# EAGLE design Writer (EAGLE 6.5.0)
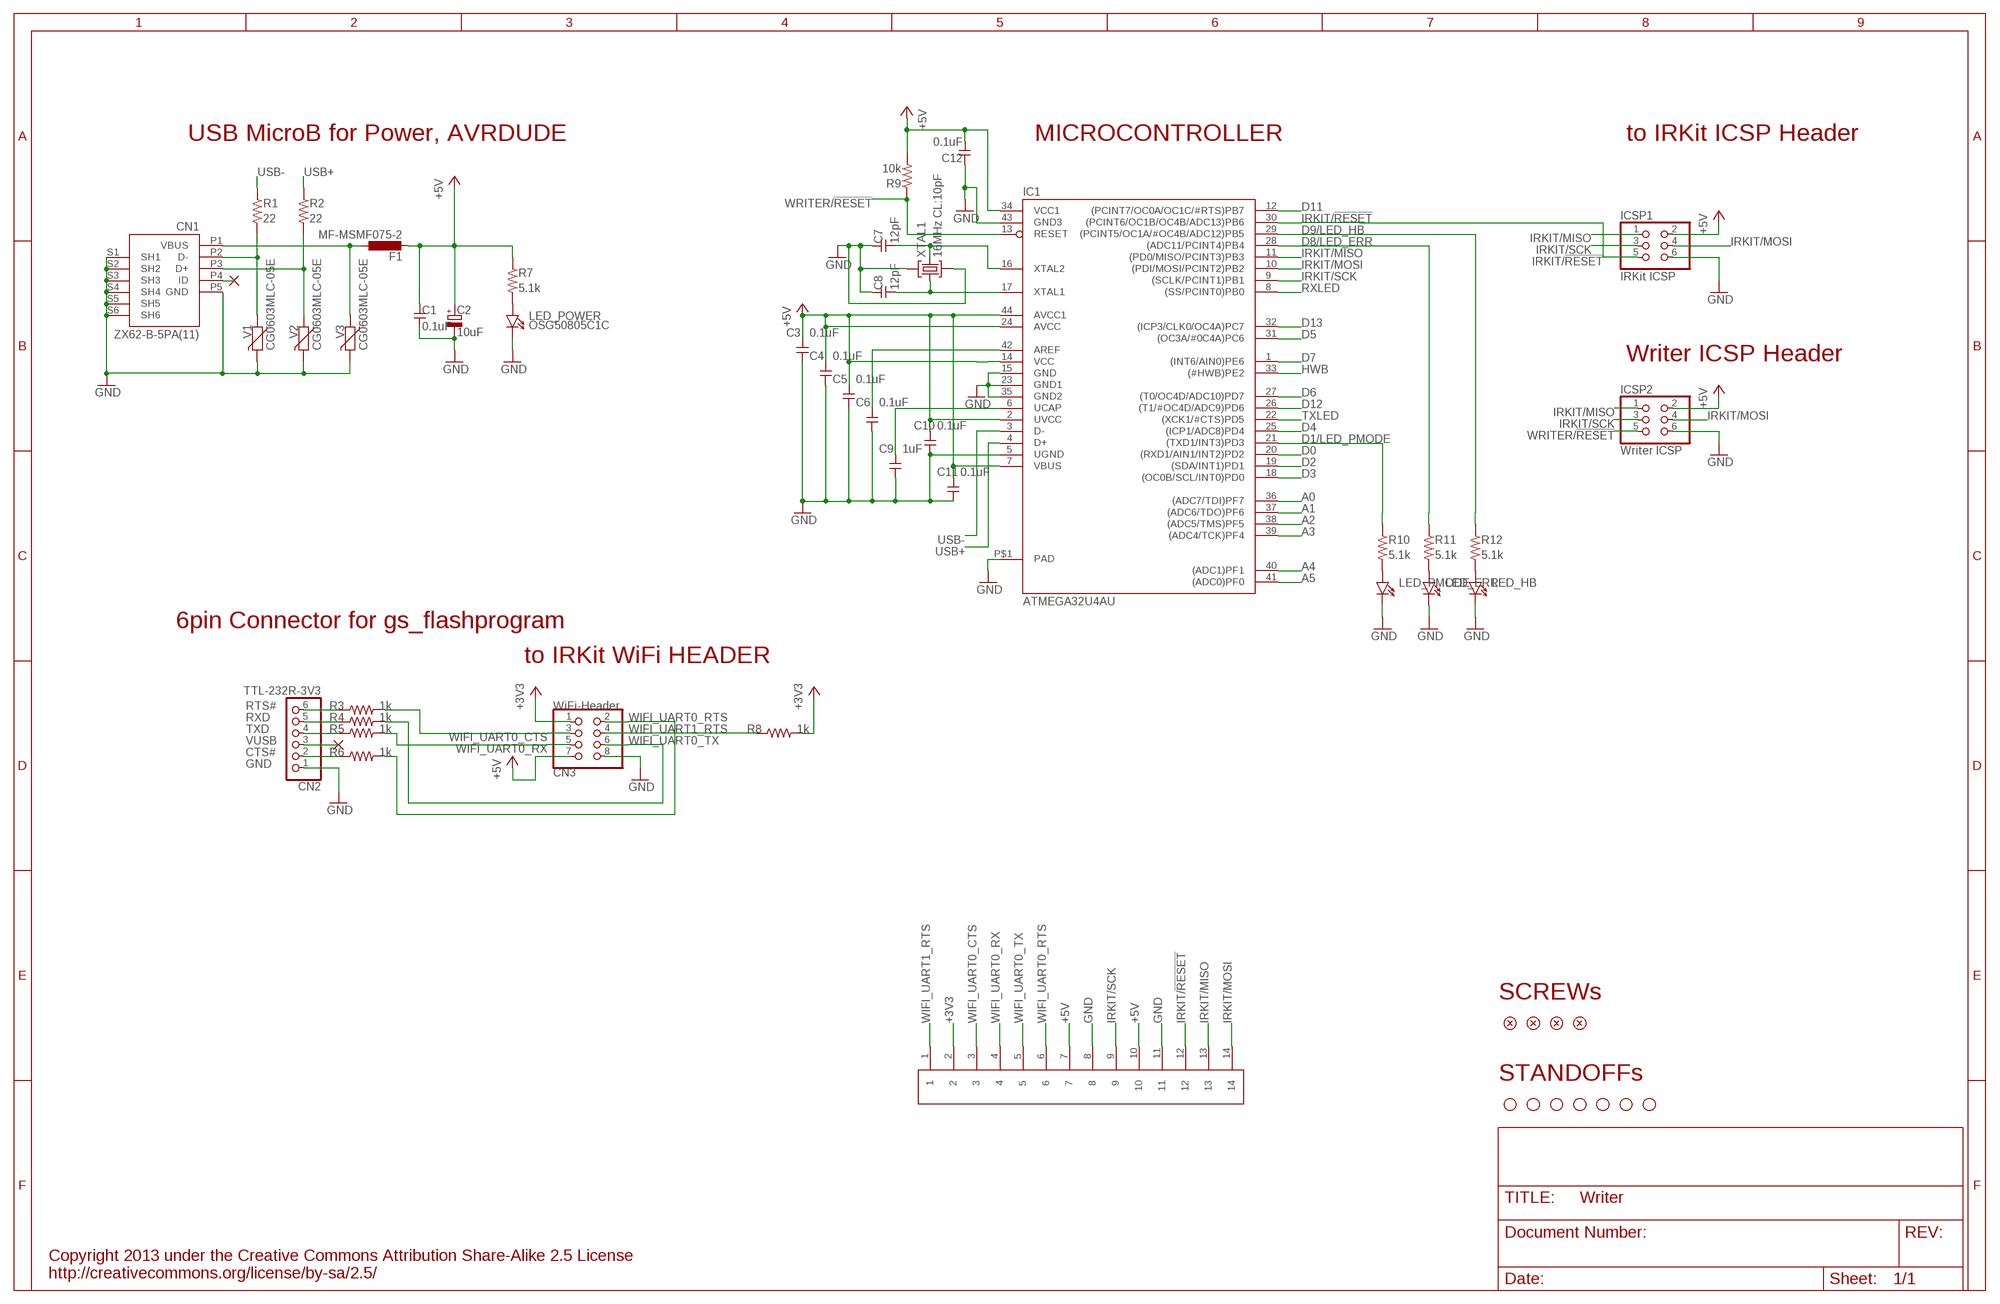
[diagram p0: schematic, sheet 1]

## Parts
C1  0.1uF  CAPACITOR2012  [SMD2012]
C2  10uF  CAPACITOR-POLPANASONIC_B  [PANASONIC_B]
C3  0.1uF  CAPACITOR2012  [SMD2012]
C4  0.1uF  CAPACITOR2012  [SMD2012]
C5  0.1uF  CAPACITOR2012  [SMD2012]
C6  0.1uF  CAPACITOR2012  [SMD2012]
C7  12pF  CAPACITOR2012  [SMD2012]
C8  12pF  CAPACITOR2012  [SMD2012]
C9  1uF  CAPACITOR2012  [SMD2012]
C10  0.1uF  CAPACITOR2012  [SMD2012]
C11  0.1uF  CAPACITOR2012  [SMD2012]
C12  0.1uF  CAPACITOR2012  [SMD2012]
CN1  ZX62-B-5PA(11)  USB-CONNECTORMICROB  [USB-MICROB]
CN2  TTL-232R-3V3  PINHD-1X6/90  [1X06/90]
CN3  WiFi-Header  PINHD-2X4/D1.1  [2X04/D1.1]
CN4  SOCKET-HEADER-7614-5002  [SOCKET-HEADER-7614-5002]
F1  MF-MSMF075-2  L-EUL1812  [L1812]
IC1  ATMEGA32U4AU  [TQFP44-PAD]
ICSP1  IRKit ICSP  PINHD-2X3/D1.1  [2X03/D1.1]
ICSP2  Writer ICSP  PINHD-2X3  [2X03]
LED_ERR  LED-2012  [LED2012]
LED_HB  LED-2012  [LED2012]
LED_PMODE  LED-2012  [LED2012]
LED_POWER  OSG50805C1C  LED-2012  [LED2012]
R1  22  RESISTOR-US2012  [SMD2012]
R2  22  RESISTOR-US2012  [SMD2012]
R3  1k  RESISTOR-US2012  [SMD2012]
R4  1k  RESISTOR-US2012  [SMD2012]
R5  1k  RESISTOR-US2012  [SMD2012]
R6  1k  RESISTOR-US2012  [SMD2012]
R7  5.1k  RESISTOR-US2012  [SMD2012]
R8  1k  RESISTOR-US2012  [SMD2012]
R9  10k  RESISTOR-US2012  [SMD2012]
R10  5.1k  RESISTOR-US2012  [SMD2012]
R11  5.1k  RESISTOR-US2012  [SMD2012]
R12  5.1k  RESISTOR-US2012  [SMD2012]
SCREW1  flat-head M3 self-tapping  SCREW  [SCREW-M3]
SCREW2  flat-head M3 self-tapping  SCREW  [SCREW-M3]
SCREW3  flat-head M3 self-tapping  SCREW  [SCREW-M3]
SCREW4  flat-head M3 self-tapping  SCREW  [SCREW-M3]
STANDOFF1  STAND-OFF  [STAND-OFF]
STANDOFF2  STAND-OFF  [STAND-OFF]
STANDOFF3  STAND-OFF  [STAND-OFF]
STANDOFF4  STAND-OFF  [STAND-OFF]
STANDOFF5  STAND-OFF  [STAND-OFF]
STANDOFF6  STAND-OFF  [STAND-OFF]
STANDOFF7  STAND-OFF  [STAND-OFF]
V1  CG0603MLC-05E  VARISTORCN0603  [CT/CN0603]
V2  CG0603MLC-05E  VARISTORCN0603  [CT/CN0603]
V3  CG0603MLC-05E  VARISTORCN0603  [CT/CN0603]
XTAL1  16MHz CL:10pF  CRYSTAL-3.2-2.5  [CRYSTAL-3.2-2.5]

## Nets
+3V3 [3.3v]: CN3.1 CN4.2 R8.2
+5V [power]: C1.1 C2.+ C3.2 C4.2 C5.2 C10.2 C11.2 C12.2 CN3.7 CN4.7 CN4.10 F1.2 IC1.2(UVCC) IC1.7(VBUS) IC1.14(VCC) IC1.24(AVCC) IC1.34(VCC1) IC1.44(AVCC1) ICSP1.2 ICSP2.2 R7.1 R9.2
A0: IC1.36((ADC7/TDI)PF7)
A1: IC1.37((ADC6/TDO)PF6)
A2: IC1.38((ADC5/TMS)PF5)
A3: IC1.39((ADC4/TCK)PF4)
A4: IC1.40((ADC1)PF1)
A5: IC1.41((ADC0)PF0)
AREF [power]: C6.2 IC1.42(AREF)
CTS#: CN2.2 R6.1
D0: IC1.20((RXD1/AIN1/INT2)PD2)
D1/LED_PMODE: IC1.21((TXD1/INT3)PD3) R10.1
D2: IC1.19((SDA/INT1)PD1)
D3: IC1.18((OC0B/SCL/INT0)PD0)
D4: IC1.25((ICP1/ADC8)PD4)
D5: IC1.31((OC3A/#0C4A)PC6)
D6: IC1.27((T0/OC4D/ADC10)PD7)
D7: IC1.1((INT6/AIN0)PE6)
D8/LED_ERR: IC1.28((ADC11/PCINT4)PB4) R11.1
D9/LED_HB: IC1.29((PCINT5/OC1A/#OC4B/ADC12)PB5) R12.1
D11: IC1.12((PCINT7/OC0A/OC1C/#RTS)PB7)
D12: IC1.26((T1/#OC4D/ADC9)PD6)
D13: IC1.32((ICP3/CLK0/OC4A)PC7)
GND [gnd]: C1.2 C2.- C3.1 C4.1 C5.1 C6.1 C7.1 C8.1 C9.1 C10.1 C11.1 C12.1 CN1.P5(GND) CN1.S1(SH1) CN1.S2(SH2) CN1.S3(SH3) CN1.S4(SH4) CN1.S5(SH5) CN1.S6(SH6) CN2.1 CN3.8 CN4.8 CN4.11 IC1.5(UGND) IC1.15(GND) IC1.23(GND1) IC1.35(GND2) IC1.43(GND3) IC1.P$1(PAD) ICSP1.6 ICSP2.6 LED_ERR.K LED_HB.K LED_PMODE.K LED_POWER.K V1.2 V2.2 V3.2 XTAL1.2(GND) XTAL1.4(GND)
HWB: IC1.33((#HWB)PE2)
IRKIT/!RESET: CN4.12 IC1.30((PCINT6/OC1B/OC4B/ADC13)PB6) ICSP1.5
IRKIT/MISO: CN4.13 IC1.11((PD0/MISO/PCINT3)PB3) ICSP1.1 ICSP2.1
IRKIT/MOSI: CN4.14 IC1.10((PDI/MOSI/PCINT2)PB2) ICSP1.4 ICSP2.4
IRKIT/SCK: CN4.9 IC1.9((SCLK/PCINT1)PB1) ICSP1.3 ICSP2.3
N$1: LED_PMODE.A R10.2
N$2: LED_ERR.A R11.2
N$3: LED_POWER.A R7.2
N$4: LED_HB.A R12.2
N$48: CN1.P2(D-) R1.2 V1.1
N$51: CN1.P3(D+) R2.2 V2.1
N$52: CN1.P1(VBUS) F1.1 V3.1
RTS#: CN2.6 R3.1
RXD: CN2.5 R4.1
RXLED: IC1.8((SS/PCINT0)PB0)
TXD: CN2.4 R5.1
TXLED: IC1.22((XCK1/#CTS)PD5)
UCAP: C9.2 IC1.6(UCAP)
USB+: IC1.4(D+) R2.1
USB-: IC1.3(D-) R1.1
USB-ID: CN1.P4(ID)
VUSB: CN2.3
WIFI_UART0_CTS: CN3.3 CN4.3 R3.2
WIFI_UART0_RTS: CN3.2 CN4.6 R6.2
WIFI_UART0_RX: CN3.5 CN4.4 R5.2
WIFI_UART0_TX: CN3.6 CN4.5 R4.2
WIFI_UART1_RTS: CN3.4 CN4.1 R8.1
WRITER/!RESET: IC1.13(RESET) ICSP2.5 R9.1
XTAL1: C8.2 IC1.17(XTAL1) XTAL1.1(C1)
XTAL2: C7.2 IC1.16(XTAL2) XTAL1.3(C2)

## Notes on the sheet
- USB MicroB for Power, AVRDUDE | MICROCONTROLLER | to IRKit ICSP Header
- Writer ICSP Header
- 6pin Connector for gs_flashprogram
- to IRKit WiFi HEADER
- SCREWs
- STANDOFFs
- Copyright 2013 under the Creative Commons Attribution Share-Alike 2.5 License
  http://creativecommons.org/license/by-sa/2.5/

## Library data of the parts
C1 C3-C12 = my:CAPACITOR: Generic Capacitor
C2 = my:CAPACITOR-POL: Generic Capacitor with Polarity
CN1 = my:USB-CONNECTOR
CN2 = my:PINHD-1X6: PIN HEADER
CN3 = my:PINHD-2X4: PIN HEADER
CN4 = my:SOCKET-HEADER: Sumitomo Standard Socket
F1 = my:L-EU: INDUCTOR, European symbol
IC1 = my:ATMEGA32U4
ICSP1 ICSP2 = my:PINHD-2X3: PIN HEADER
LED_ERR LED_HB LED_PMODE LED_POWER = my:LED: Through-hole LED
R1-R12 = my:RESISTOR-US: Generic Registor
SCREW1-SCREW4 = my:SCREW
STANDOFF1-STANDOFF7 = my:STAND-OFF: #4 Stand Off
V1-V3 = my:VARISTOR: VARISTOR
XTAL1 = my:CRYSTAL-3.2-2.5

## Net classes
0 default: width 0.254 mm
1 power: width 0.406 mm
2 ir-power: width 0.813 mm
3 gnd: width 0.406 mm
4 3.3v: width 0.406 mm

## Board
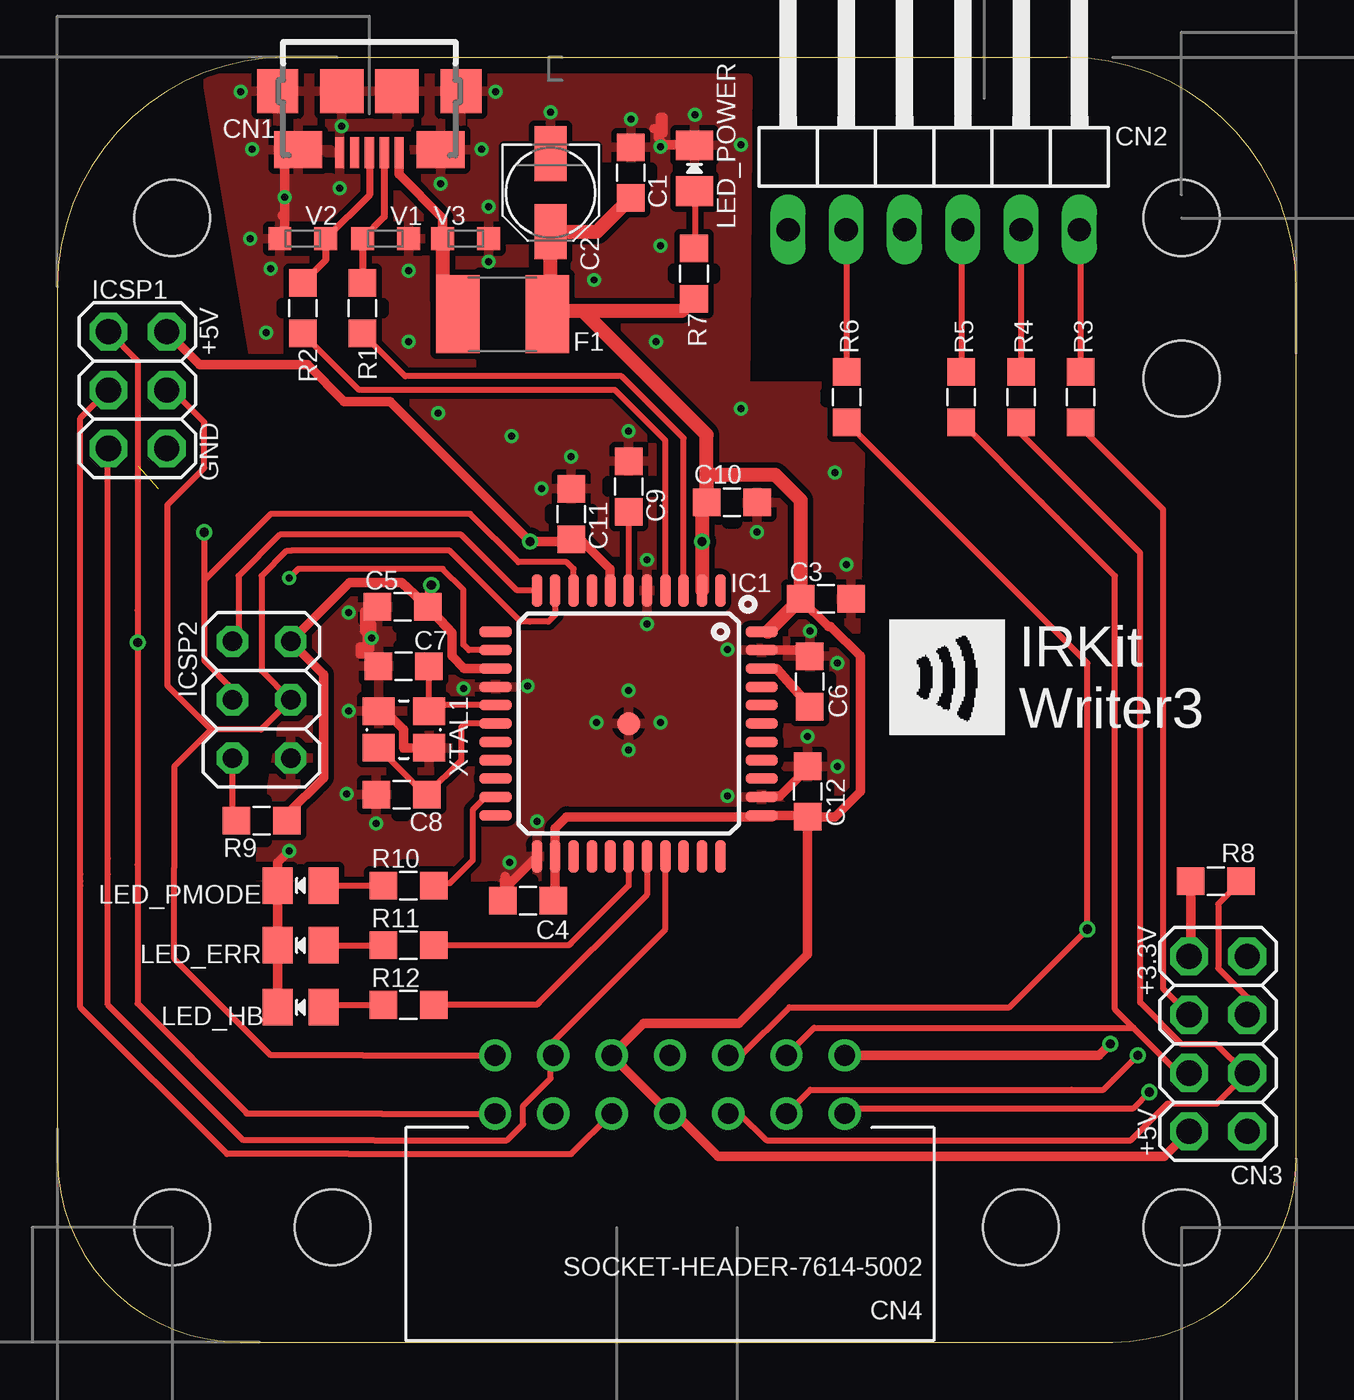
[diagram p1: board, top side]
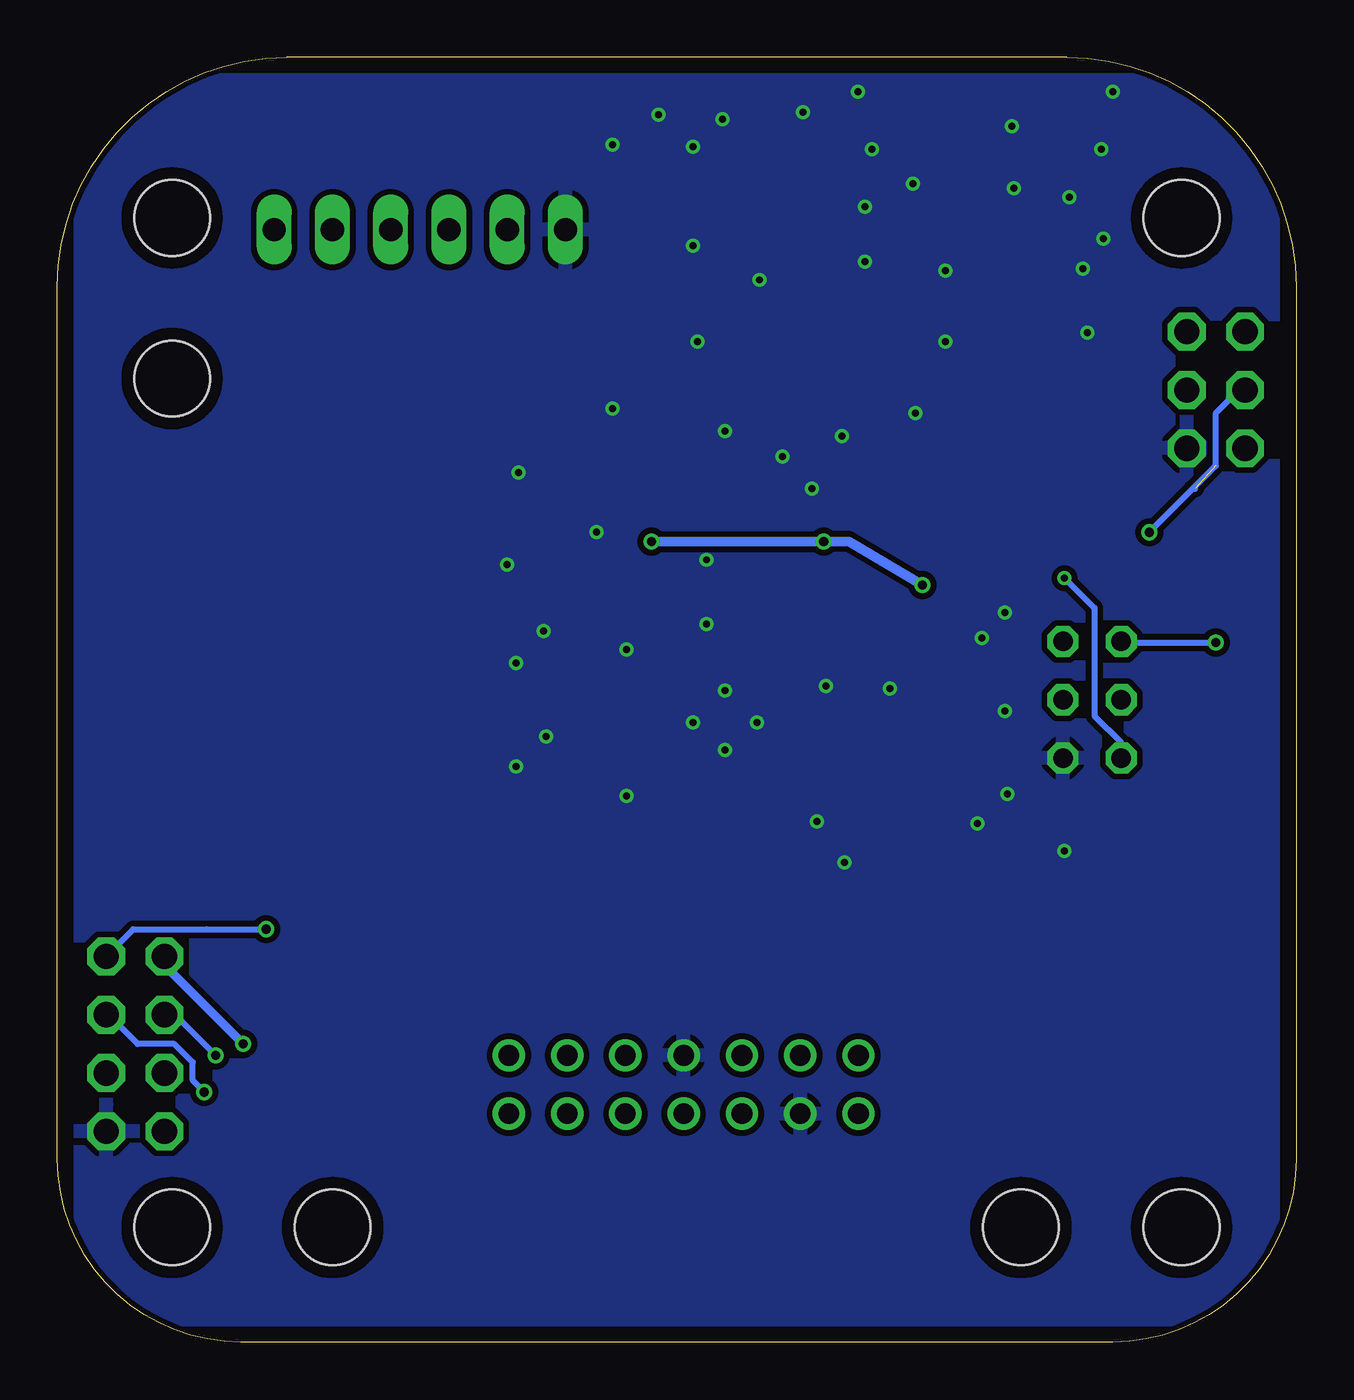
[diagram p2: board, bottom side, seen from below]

Size 54 x 56 mm. Coordinates in mm from the lower left corner, seen from the top.
Outline: 8,0 46,0 arc90 54,8 54,17.5 54,34.8 54,46 arc90 44,56 34.1,56 34,56 20,56 10,56 arc90 0,46 0,8 arc90 8,0
Copper layers (1*16): Top 0.035mm / dielectric 1.5mm / Bottom 0.035mm
Design rules "Fusion_eagle_rule_v1.1": minimum track width 6mil, minimum drill 12mil, track to track 6mil, track to pad 6mil, pad to pad 6mil, via to via 6mil, smd to smd 0mil, copper to edge 10mil, drill to drill 10mil, minimum pad ring 10mil, minimum via ring 6mil, stop-mask expansion 2mil, vias tented up to drill 100mil, thermal gap 10mil

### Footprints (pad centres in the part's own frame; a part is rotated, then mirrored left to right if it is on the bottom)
SMD2012 = smd 1.2 x 1.2: 1 -1.1,0; 2 1.1,0
PANASONIC_B = smd 2.4 x 1.4: + 1.7,0; - -1.7,0
USB-MICROB = smd 0.4 x 1.35: P1 -1.3,2.675; P2 -0.65,2.675; P3 0,2.675; P4 0.65,2.675; P5 1.3,2.675 | smd 1.8 x 1.9: S1 -4,0; S2 4,0 | smd 2.1 x 1.6: S3 -3.1,2.55; S4 3.1,2.55 | smd 1.9 x 1.9: S5 -1.2,0; S6 1.2,0
1X06/90 = drill 1.016 long: 1 -6.35,-3.81; 2 -3.81,-3.81; 3 -1.27,-3.81; 4 1.27,-3.81; 5 3.81,-3.81; 6 6.35,-3.81
2X04/D1.1 = drill 1.1 octagon: 1 -3.81,-1.27; 2 -3.81,1.27; 3 -1.27,-1.27; 4 -1.27,1.27; 5 1.27,-1.27; 6 1.27,1.27; 7 3.81,-1.27; 8 3.81,1.27
SOCKET-HEADER-7614-5002 = drill 0.9: 1 -7.62,2.54; 2 -7.62,0; 3 -5.08,2.54; 4 -5.08,0; 5 -2.54,2.54; 6 -2.54,0; 7 0,2.54; 8 0,0; 9 2.54,2.54; 10 2.54,0; 11 5.08,2.54; 12 5.08,0; 13 7.62,2.54; 14 7.62,0
L1812 = smd 1.9 x 3.4: 1 -1.95,0; 2 1.95,0
TQFP44-PAD = smd 1.4 x 0.45: 1 -5.8,4; 2 -5.8,3.2; 3 -5.8,2.4; 4 -5.8,1.6; 5 -5.8,0.8; 6 -5.8,0; 7 -5.8,-0.8; 8 -5.8,-1.6; 9 -5.8,-2.4; 10 -5.8,-3.2; 11 -5.8,-4; 23 5.8,-4; 24 5.8,-3.2; 25 5.8,-2.4; 26 5.8,-1.6; 27 5.8,-0.8; 28 5.8,0; 29 5.8,0.8; 30 5.8,1.6; 31 5.8,2.4; 32 5.8,3.2; 33 5.8,4 | smd 0.45 x 1.4: 12 -4,-5.8; 13 -3.2,-5.8; 14 -2.4,-5.8; 15 -1.6,-5.8; 16 -0.8,-5.8; 17 0,-5.8; 18 0.8,-5.8; 19 1.6,-5.8; 20 2.4,-5.8; 21 3.2,-5.8; 22 4,-5.8; 34 4,5.8; 35 3.2,5.8; 36 2.4,5.8; 37 1.6,5.8; 38 0.8,5.8; 39 0,5.8; 40 -0.8,5.8; 41 -1.6,5.8; 42 -2.4,5.8; 43 -3.2,5.8; 44 -4,5.8 | smd 1 x 1: P$1 0,0
2X03/D1.1 = drill 1.1 octagon: 1 -2.54,-1.27; 2 -2.54,1.27; 3 0,-1.27; 4 0,1.27; 5 2.54,-1.27; 6 2.54,1.27
2X03 = drill 0.85 octagon: 1 -2.54,-1.27; 2 -2.54,1.27; 3 0,-1.27; 4 0,1.27; 5 2.54,-1.27; 6 2.54,1.27
LED2012 = smd 1.3 x 1.6: A -1,0; K 1,0
STAND-OFF = hole 3.302: 0,0
CT/CN0603 = smd 1 x 1: 1 -1,0; 2 1,0
CRYSTAL-3.2-2.5 = smd 1.4 x 1.2: 1 -1.1,-0.8; 2 1.1,-0.8; 3 1.1,0.8; 4 -1.1,0.8

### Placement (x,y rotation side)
C1  25,50.97 90 top
C2  21.5,50.1 270 top
C3  33.5,32.4 180 top
C4  20.51,19.25 0 top
C5  15.05,32.05 0 top
C6  32.8,28.8 270 top
C7  15.1,29.46 0 top
C8  15,23.86 0 top
C9  24.9,37.3 270 top
C10  29.4,36.6 180 top
C11  22.4,36.1 270 top
C12  32.7,24 270 top
CN1  13.6,54.52 180 top
CN2  38.2,52.3 0 top
CN3  50.6,13 270 top
CN4  26.7,12.5 180 top
F1  19.4,44.8 0 top
IC1  24.9,26.96 270 top
ICSP1  3.5,41.5 270 top
ICSP2  8.9,28 270 top
LED_ERR  10.6,17.3 180 top
LED_HB  10.6,14.6 180 top
LED_PMODE  10.6,19.9 180 top
LED_POWER  27.77,51.16 90 top
R1  13.3,45.06 90 top
R2  10.7,45.06 90 top
R3  44.6,41.2 270 top
R4  42,41.2 270 top
R5  39.4,41.2 270 top
R6  34.4,41.2 270 top
R7  27.75,46.58 90 top
R8  50.5,20.1 180 top
R9  8.9,22.73 0 top
R10  15.3,19.9 180 top
R11  15.3,17.3 180 top
R12  15.3,14.7 180 top
SCREW1  not placed on the board
SCREW2  not placed on the board
SCREW3  not placed on the board
SCREW4  not placed on the board
STANDOFF1  49,5 0 top
STANDOFF2  5,5 0 top
STANDOFF3  49,49 0 top
STANDOFF4  5,49 0 top
STANDOFF5  12,5 0 top
STANDOFF6  42,5 0 top
STANDOFF7  49,42 0 top
U$1  [IRKIT-LOGO]  36.3,26.5 0 top
V1  14.3,48.1 0 top
V2  10.7,48.1 180 top
V3  17.8,48.1 0 top
XTAL1  15.1,26.7 0 top

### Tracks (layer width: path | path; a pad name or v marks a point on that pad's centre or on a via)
+3V3  (via drill 0.4)
  Top 0.406: R8.2 49.4,16.9 CN3.1 | CN4.2 45.4,12.5 v45.9,13
  Bottom 0.406: v45.9,13 49.33,16.43 CN3.1
+5V  (via drill 0.4)
  Top 0.406: v20.6,34.9 22.5,34.9 | 20.6,34.8 v20.6,34.9 | v20.6,34.9 14.5,41 12.5,41 10.9,42.6 9.9,42.6 6.21,42.6 ICSP1.2 | C5.2 15,33.1 13.3,33.1 12.73,33.1 ICSP2.2 11.6,29.11 11.6,24.6 10,23 R9.2 | v16.3,33 16.25,32.95 C5.2 | C5.2 17.2,30.9 17.2,29.9 17.74,29.36 IC1.14 | 49.33,9.13 CN3.7 48.24,8.1 28.8,8.1 26.94,9.96 CN4.7 CN4.10 25.56,13.9 29.6,13.9 29.7,13.9 32.7,16.9 C12.2 | IC1.7 24.1,33.7 22.9,34.9 22.5,34.9 | 22.5,34.9 C11.2 | IC1.44 30.96,30.96 | IC1.34 31.2,22.96 | 31.2,22.96 32.64,22.96 C12.2 | C12.2 33.9,22.9 35,24 35,29.9 33.7,31.2 33.6,31.2 C3.2 | 31.2,22.96 31.14,22.9 22.2,22.9 21.7,22.4 IC1.24 21.7,19.34 C4.2
  Top 0.61: IC1.2 v28.1,34.9 28.1,36.4 C10.2 28.3,37.8 | 30.96,30.96 C3.2 32.4,36.7 31.3,37.8 28.3,37.8 | F1.2 21.5,44.95 | 21.5,44.95 C2.+ 23.52,48.4 C1.1 | 21.5,44.95 22.9,44.95 | 22.9,44.95 27.23,44.95 R7.1 | 28.3,37.8 28.3,39.55 22.9,44.95 | 28.3,37.8 28.3,36.5
  Top 0.813: 21.35,48.25 C2.+ | 27.73,45.5 R7.1
  Bottom 0.406: v28.1,34.9 v20.6,34.9 19.5,34.9 v16.3,33
AREF
  Top 0.406: IC1.42 31.34,29.36 C6.2
CTS#
  Top 0.254: R6.1 34.4,48.4 CN2.2
D1/LED_PMODE
  Top 0.254: IC1.21 19.1,23.7 18.6,23.7 18.1,23.2 18.1,21 17.1,20 16.5,20 R10.1
D8/LED_ERR
  Top 0.254: IC1.28 24.9,21.1 24.9,19.9 22.4,17.4 22.3,17.3 R11.1
D9/LED_HB
  Top 0.254: IC1.29 25.7,21.1 25.7,19.5 21,14.8 20.9,14.7 R12.1
GND  (via drill 0.3)
  Top 0.406: LED_POWER.K 27.7,52.2 26.4,52.2 26.3,52.3 26.3,52.4 26.2,52.5 26.2,52.8 26.3,52.9 26.3,53.4 26.4,53.4 26.4,52.7 26.3,52.7 26.3,52.8 26.2,52.9 26,52.9 | 19.51,20.3 19.5,20.1 19.6,20 19.6,19.8 19.7,19.8 19.7,20.1 19.6,20.1 19.5,20 19.5,19.3 C4.1 19.41,19.68 IC1.23 | XTAL1.2 15.1,25.9 15.1,26.7 14.4,27.4 XTAL1.4 | V2.2 9.9,48.3 9.9,49.1 | 9.9,49.1 9.9,51.3 10.5,51.9 | 10.5,51.9 CN1.S4 10.5,51.9 | v13.7,30.7 13.7,31.3 13.5,31.3 13.5,31 13.6,30.9 13.6,30.2 13.5,30.1 13.4,30.2 13.4,30.3 13.2,30.3 13.2,30 13.3,30 13.5,30.2 13.5,30.9 13.4,31 13.4,31.5 13.4,31.85 | 10.5,51.9 10.5,51.78 | 9.8,49.1 9.9,49.1 | IC1.43 32.46,30.16 C6.1 | IC1.35 30.74,23.8 31.5,23.8 32.7,25 C12.1 | LED_HB.K 9.6,17.1 LED_ERR.K LED_PMODE.K 9.6,20.1 9.6,20.9 v10.1,21.4
  other vias: 22.4,38.6 12.3,50.3 15.3,46.7 18.8,49.5 34.4,33.9 9.9,49.9 8.5,52 19.1,54.5 18.5,52 16.7,50.5 15.3,43.6 21.5,53.6 25,53.3 26.3,52.1 26.3,47.8 30.5,35.3 24.9,39.7 16.6,40.5 23.4,46.3 12.7,31.8 12.7,27.5 12.6,23.9 19.7,20.9 20.5,28.6 20.9,22.7 24.9,25.8 26.3,27 23.5,27 24.9,28.4 25.7,31.3 29.2,30.2 29.2,23.8 34,25.1 32.7,26.4 34,29.6 29.8,40.7 21.1,37.2 33.9,37.9 19.8,39.5 26.1,43.6 29.8,52.2 27.8,53.5 25.7,34.1 9.1,44 8,54.5 12.4,53 8.4,48.1 9.3,46.8 32.8,31 18.8,47.1 17.7,28.5 13.9,22.6
  pour Bottom (isolate 0.254): 1,1 1,55 53,55 53,1
  pour Top (isolate 0.254): 12.2,41.6 35.1,41.7 34.5,20.2 8.7,20.3
  pour Top (isolate 0.254): 30,41.4 8.8,41.5 6.5,55.1 30.1,55.1
IRKIT/!RESET
  Top 0.254: 2.2,20.4 2.2,21.1 | 2.2,21.1 2.2,38.93 2.3,39 ICSP1.5 | IC1.30 26.5,18 21.62,13.12 CN4.12 21.5,12.38 21.5,11.5 20.3,10.3 20.3,9.5 19.6,8.8 13.8,8.8 8.1,8.8 2.2,14.7 2.2,21.1
IRKIT/MISO  (via drill 0.4)
  Top 0.254: CN4.13 14.14,9.96 8.3,9.96 | IC1.11 20.04,32.76 17.6,35.2 9.7,35.2 7.9,33.4 7.9,30.81 ICSP2.1 | 8.3,9.96 8.24,9.96 | ICSP1.1 3.5,42.77 3.5,31.9 v3.5,30.5 3.5,20.8 3.5,14.76 8.3,9.96
  Bottom 0.254: ICSP2.1 7.59,30.5 v3.5,30.5
IRKIT/MOSI
  Top 0.254: IC1.10 21.7,31.7 21.4,31.4 20.6,31.4 20.2,31.4 18.1,33.5 17.1,34.5 10.2,34.5 10,34.5 8.9,33.4 8.9,29.27 ICSP2.4 | 10.17,28.13 ICSP2.4 | ICSP2.4 8.97,26.8 8.87,26.7 6.7,26.7 | CN4.14 13.3,12.5 9.3,12.5 5.2,16.6 5.1,16.7 5.1,20.7 5.1,25.1 6.7,26.7 | 6.7,26.7 4.8,28.6 4.8,36.5 6.4,38.1 6.4,40.1 5,41.5 ICSP1.4
IRKIT/SCK  (via drill 0.4)  (1 unrouted)
  Top 0.254: 1,20.1 1,20.4 | 1,20.4 1,40.27 ICSP1.3 | 1,20.4 1,19.9 1,14.6 7.4,8.2 12.7,8.2 19.7,8.2 22.4,8.2 CN4.9 | IC1.9 22.5,33.7 22.2,34 20.1,34 18,36.1 9.3,36.1 6.4,33.2 6.4,33 | 6.4,33 6.4,29.7 7.63,28.47 ICSP2.3 | v6.4,35.3 6.4,33
  Bottom 0.254: 4.4,37.2 4.5,37.2 | ICSP1.3 2.3,41.5 2.4,41.5 2.5,41.5 3.5,40.5 3.5,38.2 v6.4,35.3
N$1
  Top 0.254: LED_PMODE.A R10.2
N$2
  Top 0.254: LED_ERR.A R11.2
N$3
  Top 0.254: R7.2 27.8,47.7 27.8,50.1 LED_POWER.A
N$4
  Top 0.254: 11.6,14.7 R12.2
  Top 0.406: LED_HB.A 11.6,14.7
N$48
  Top 0.305: CN1.P2 14.25,49.05 V1.1 R1.2
N$51
  Top 0.305: CN1.P3 13.6,50 V2.1 11.7,47.16 R2.2
N$52
  Top 0.406: CN1.P1 14.9,50.9 16.8,49 V3.1
  Top 0.61: V3.1 16.8,45.45 F1.1
RTS#
  Top 0.254: R3.1 44.6,48.4 CN2.6
RXD
  Top 0.254: R4.1 42,48.4 CN2.5
TXD
  Top 0.254: R5.1 39.4,48.4 CN2.4
UCAP
  Top 0.254: C9.2 IC1.6
USB+
  Top 0.254: IC1.4 26.5,39.3 24.3,41.5 13.16,41.5 R2.1
USB-
  Top 0.254: IC1.3 27.3,39.4 24.6,42.1 15.16,42.1 R1.1
WIFI_UART0_CTS  (via drill 0.4)
  Top 0.254: CN3.3 49.3,14.3 48.2,15.4 48.2,36.3 44.6,39.9 R3.2 | CN4.3 32.82,11 44.2,11 45.6,11 v47.1,12.5
  Bottom 0.254: v47.1,12.5 48.87,14.27 CN3.3
WIFI_UART0_RTS  (via drill 0.4)
  Top 0.254: 51.9,16.8 CN3.2 | R6.2 44.9,29.6 v44.9,18 41.5,14.6 31.9,14.6 29.8,12.5 CN4.6
  Bottom 0.254: v44.9,18 47.5,18 50.7,18 50.7,17.98 CN3.2
WIFI_UART0_RX
  Top 0.254: R5.2 42.9,36.6 46.1,33.4 46.1,14.5 46.9,13.7 | CN3.5 49.3,11.8 48.8,11.8 46.9,13.7 | CN4.4 32.98,13.7 46.9,13.7
WIFI_UART0_TX
  Top 0.254: R4.2 42,39.6 47.2,34.4 47.2,14.8 49,13 50.5,13 51.77,11.73 CN3.6 50.54,10.4 48.4,10.4 46.8,8.8 30.9,8.8 29.74,9.96 CN4.5
WIFI_UART1_RTS  (via drill 0.4)
  Top 0.254: R8.1 50.9,19.4 50.6,19.1 50.6,16.3 51.87,15.03 CN3.4 51.8,14.3 | CN4.1 34.56,10.2 46.9,10.2 v47.6,10.9
  Bottom 0.254: CN3.4 51.77,14.27 50.5,13 48.9,13 48.1,12.2 48.1,11.4 v47.6,10.9
WRITER/!RESET  (via drill 0.3)
  Top 0.254: ICSP2.5 7.63,23.2 R9.1 | IC1.13 17.94,30.16 17.7,30.4 17.7,32.8 16.8,33.7 12.5,33.7 10.5,33.7 v10.1,33.3
  Bottom 0.254: v10.1,33.3 8.8,32 8.8,27.3 7.63,26.13 ICSP2.5
XTAL1
  Top 0.254: IC1.17 17.76,26.96 17.6,26.8 17.6,25.36 C8.2 16.04,23.86 XTAL1.1
XTAL2
  Top 0.254: C7.2 16.2,29.5 XTAL1.3 16.46,27.76 IC1.16

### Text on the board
tPlace: +5V | GND | IRKit / Writer3 | +3.3V | +5V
